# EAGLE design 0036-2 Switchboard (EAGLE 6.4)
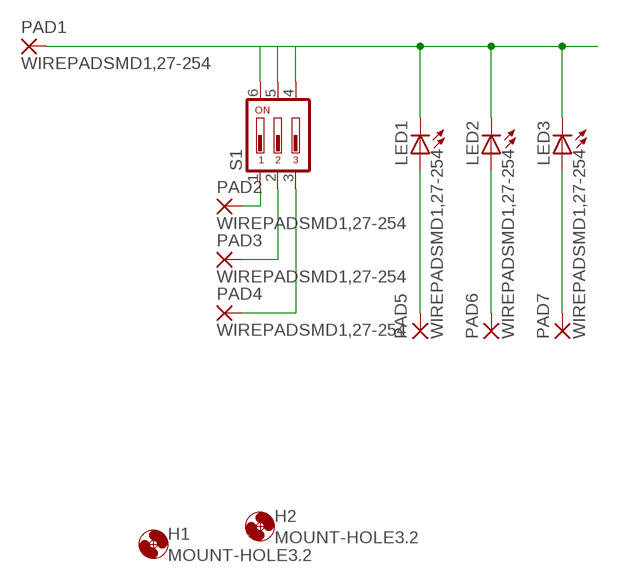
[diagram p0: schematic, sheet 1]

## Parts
H1  MOUNT-HOLE3.2  [3,2]
H2  MOUNT-HOLE3.2  [3,2]
LED1  LED5MM  [LED5MM]
LED2  LED5MM  [LED5MM]
LED3  LED5MM  [LED5MM]
PAD1  WIREPADSMD1,27-254  [SMD1,27-2,54]
PAD2  WIREPADSMD1,27-254  [SMD1,27-2,54]
PAD3  WIREPADSMD1,27-254  [SMD1,27-2,54]
PAD4  WIREPADSMD1,27-254  [SMD1,27-2,54]
PAD5  WIREPADSMD1,27-254  [SMD1,27-2,54]
PAD6  WIREPADSMD1,27-254  [SMD1,27-2,54]
PAD7  WIREPADSMD1,27-254  [SMD1,27-2,54]
S1  DIP03YL  [DIP03YL]

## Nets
N$1: LED1.K(C) LED2.K(C) LED3.K(C) PAD1.1(P) S1.4 S1.5 S1.6
N$2: PAD2.1(P) S1.1
N$3: PAD3.1(P) S1.2
N$4: PAD4.1(P) S1.3
N$5: LED3.A PAD7.1(P)
N$6: LED2.A PAD6.1(P)
N$7: LED1.A PAD5.1(P)

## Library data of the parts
H1 H2 = holes:MOUNT-HOLE: MOUNTING HOLE with drill center marker
LED1-LED3 = led:LED: LED
PAD1-PAD7 = wirepad:WIREPAD: Wire PAD connect wire on PCB
S1 = switch-dil:DIP03YL: DIL/CODE SWITCH; OC_FARNELL: unknown; OC_NEWARK: unknown

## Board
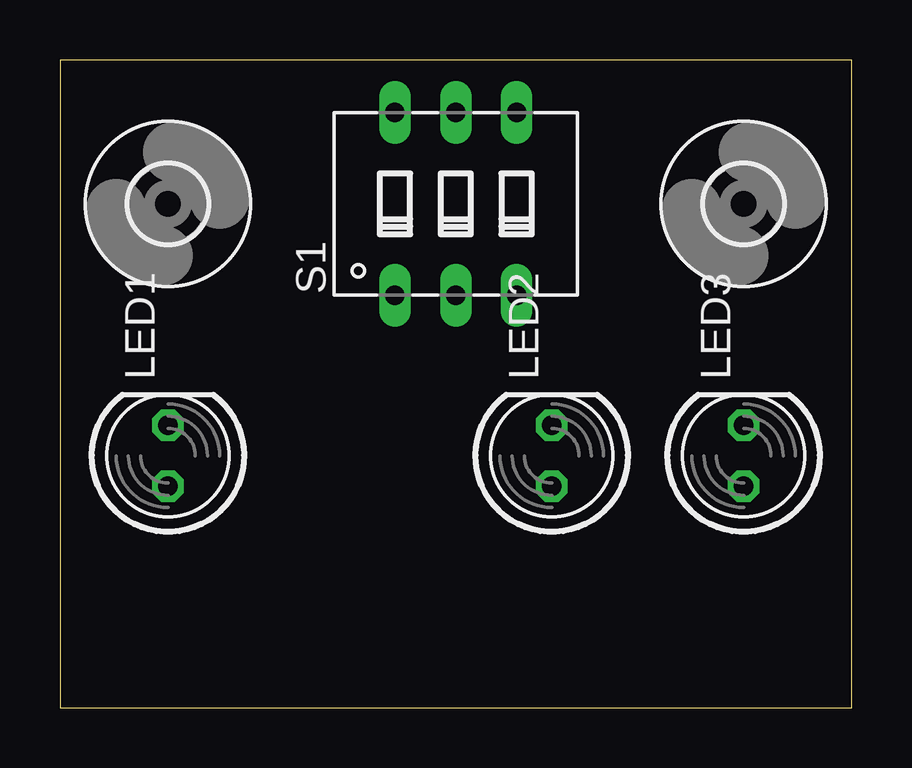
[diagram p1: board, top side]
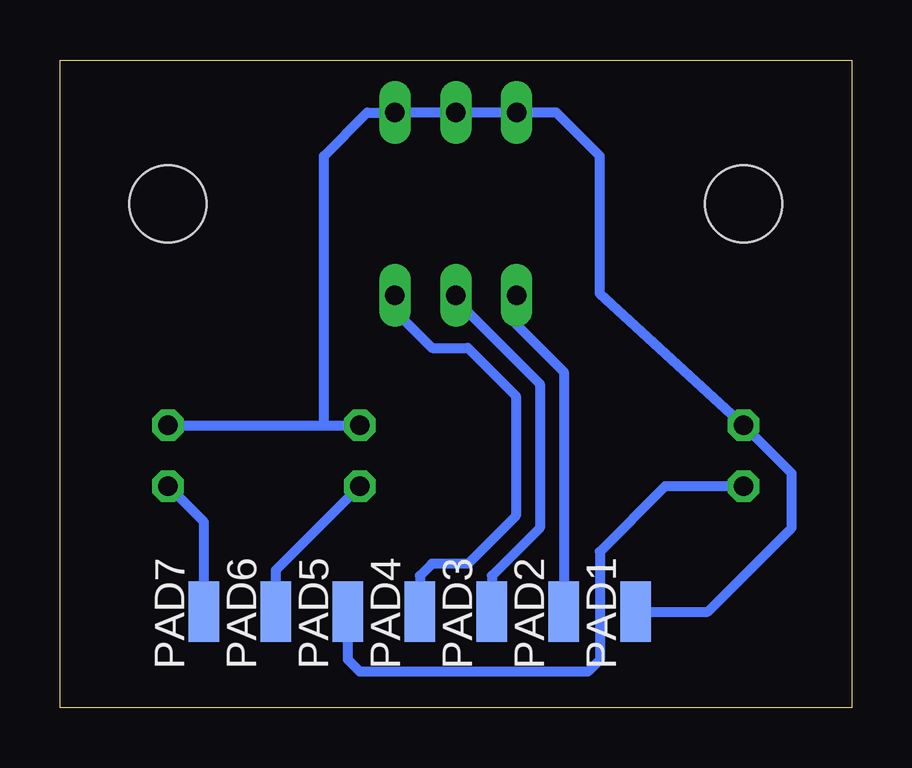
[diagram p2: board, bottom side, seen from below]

Size 33 x 27 mm. Coordinates in mm from the lower left corner, seen from the top.
Outline: 0,0 33,0 33,27 0,27 0,0
Copper layers (1*16): Top 0.035mm / dielectric 1.5mm / Bottom 0.035mm
Design rules "default": minimum track width 10mil, minimum drill 24mil, track to track 8mil, track to pad 8mil, pad to pad 8mil, via to via 8mil, smd to smd 8mil, copper to edge 40mil, drill to drill 8mil, minimum pad ring 10mil, minimum via ring 8mil, stop-mask expansion 4mil, vias tented up to drill 0mil, thermal gap 10mil

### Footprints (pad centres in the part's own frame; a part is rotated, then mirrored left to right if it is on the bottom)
3,2 = hole 3.2: 0,0
LED5MM = drill 0.813 octagon: A -1.27,0; K 1.27,0
SMD1,27-2,54 = smd 1.27 x 2.54: 1 0,0
DIP03YL = drill 0.813 long: 1 -2.54,-3.81; 2 0,-3.81; 3 2.54,-3.81; 4 2.54,3.81; 5 0,3.81; 6 -2.54,3.81

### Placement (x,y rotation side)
H1  4.5,21 0 top
H2  28.5,21 0 top
LED1  4.5,10.5 90 top
LED2  20.5,10.5 90 top
LED3  28.5,10.5 90 top
PAD1  9,4 0 bottom
PAD2  12,4 0 bottom
PAD3  15,4 0 bottom
PAD4  18,4 0 bottom
PAD5  21,4 0 bottom
PAD6  24,4 0 bottom
PAD7  27,4 0 bottom
S1  16.5,21 0 top

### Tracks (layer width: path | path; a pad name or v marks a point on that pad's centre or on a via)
N$1
  Bottom 0.406: LED3.K 22,11.77 | 22,11.77 22,23 20.19,24.81 S1.4 S1.5 S1.6 12.31,24.81 10.5,23 10.5,17.27 LED1.K 2.5,9.77 2.5,7.5 6,4 PAD1.1 | 22,11.77 LED2.K
N$2
  Bottom 0.406: S1.1 13.96,15.96 12,14 PAD2.1
N$3
  Bottom 0.406: S1.2 16.5,17 13,13.5 13,7.5 15,5.5 PAD3.1
N$4
  Bottom 0.406: S1.3 19.04,16.54 17.5,15 16,15 14,13 14,8 16,6 17.5,6 18,5.5 PAD4.1
N$5
  Bottom 0.406: PAD7.1 27,7.73 LED3.A
N$6
  Bottom 0.406: PAD6.1 24,5.73 LED2.A
N$7
  Bottom 0.406: PAD5.1 21,2 20.5,1.5 11,1.5 10.5,2 10.5,6.5 7.77,9.23 LED1.A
